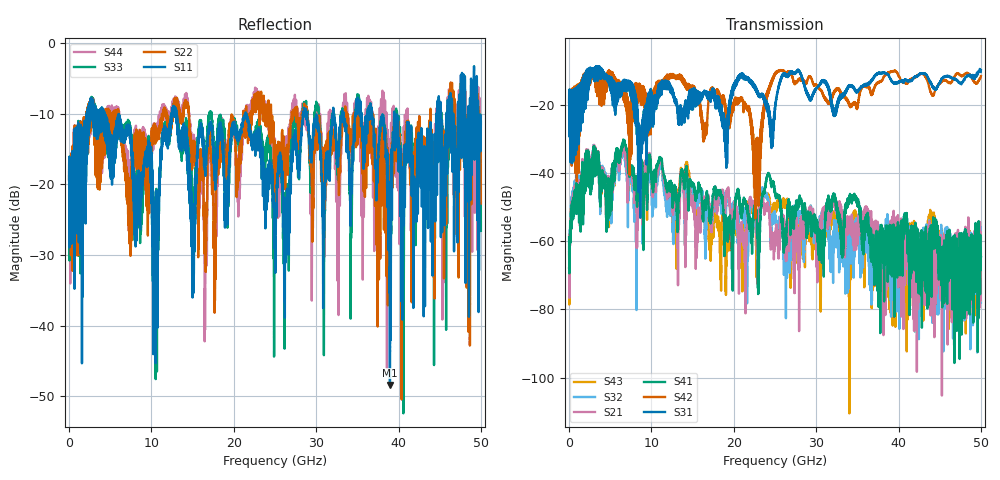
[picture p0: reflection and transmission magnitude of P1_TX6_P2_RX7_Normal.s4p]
!Keysight Technologies,N5225B,MY57041031,A.13.20.10
!Date: Friday, May 31, 2019 11:38:57
!Correction: S11(Full 4 Port(1,2,3,4))
!S12(Full 4 Port(1,2,3,4))
!S13(Full 4 Port(1,2,3,4))
!S14(Full 4 Port(1,2,3,4))
!S21(Full 4 Port(1,2,3,4))
!S22(Full 4 Port(1,2,3,4))
!S23(Full 4 Port(1,2,3,4))
!S24(Full 4 Port(1,2,3,4))
!S31(Full 4 Port(1,2,3,4))
!S32(Full 4 Port(1,2,3,4))
!S33(Full 4 Port(1,2,3,4))
!S34(Full 4 Port(1,2,3,4))
!S41(Full 4 Port(1,2,3,4))
!S42(Full 4 Port(1,2,3,4))
!S43(Full 4 Port(1,2,3,4))
!S44(Full 4 Port(1,2,3,4))
!S4P File: Measurements: <S11,S12,S13,S14>,
!<S21,S22,S23,S24>,
!<S31,S32,S33,S34>,
!<S41,S42,S43,S44>:
# Hz S  dB  R 50.0
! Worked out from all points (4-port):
!   5000 points, 10 MHz to 50 GHz, reference 50 ohm
!   strongest paths, dB at 10 MHz, 12.51 GHz, 25.01 GHz, 37.51 GHz, 50 GHz:
!     S31: -19.3, -15.5, -21.6, -10.8, -9.9
!     S42: -19.4, -12.1, -11.3, -13.6, -11.7
!     S41: -58.8, -45.4, -45.6, -63.7, -64.5
!     S21: -68.0, -45.9, -58.5, -56.8, -59.1
!     S32: -61.9, -48.6, -52.3, -62.8, -77.9
!     S43: -63.3, -51.1, -48.8, -58.5, -63.8
!   lowest |S11| = -48.4 dB at 38.96 GHz (marker M1), VSWR 1.01, Z = 50.3 + j0.217 ohm
!   |S11| at or under -10 dB: 4.286 GHz to 12.47 GHz (8.179 GHz wide, 97.6 % of centre); 13.02 GHz to 21.43 GHz (8.402 GHz wide, 48.8 % of centre); 21.46 GHz to 28.42 GHz (6.96 GHz wide, 27.9 % of centre)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
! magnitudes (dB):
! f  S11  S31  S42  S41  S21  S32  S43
! 10 MHz  -19.3  -19.3  -19.4  -58.8  -68.0  -61.9  -63.3
! 6.54 GHz  -13.8  -15.9  -17.2  -30.9  -32.9  -33.5  -31.8
! 16.54 GHz  -18.8  -16.7  -26.2  -48.8  -48.3  -63.8  -56.3
! 22.8 GHz  -13.7  -16.3  -36.9  -54.2  -62.6  -54.3  -64.9
! 25.28 GHz  -19.0  -16.7  -10.3  -46.5  -57.4  -57.6  -50.3
! 38.96 GHz  -48.4  -12.3  -10.5  -58.0  -55.9  -61.6  -62.8
! 50 GHz  -11.1  -9.9  -11.7  -64.5  -59.1  -77.9  -63.8
